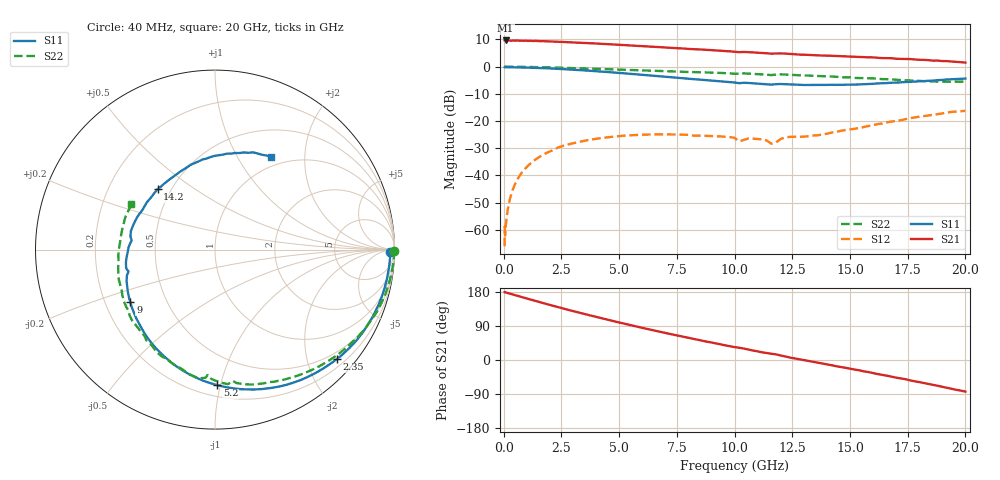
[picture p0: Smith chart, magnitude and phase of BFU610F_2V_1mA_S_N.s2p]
! Filename:  P:\Prog\Test\Noise\ATS_data\Testdata_Net\SplitFiles\BFU610_2W_A5_HighFreq_2V_1mA_D.s2p
! Date/Time: Wed 10/Aug/2011 16:55:42
! BFU610_2W_A5_HighFreq_2V_1mA_10mA_Bias1_R.s2p
! MDIF S-parameter v. bias file
! BFU610_2W_A5_HighFreq_2V_1mA_10mA
! Date/time Mon Aug 08 14:20:39 2011
! bias mode 1
! bias variable = I_out
! VAR bias_var= 1
! VAR V_out= 2.0002
! VAR I_out= 1.0000
! VAR V_in= 0.8491
! VAR I_in= 0.0074
! Device data file deembeded for feedlines and parallel
! Original file: \SplitFiles\BFU610_2W_A5_HighFreq_2V_1mA_R.s2p
! Feed-files: PR003V01_101208_Feed1.s2p, PR003V01_101208_Feed2.s2p
! Parallel-file: PR003V01_101208_Par.s2p
# MHz S MA R 50
!  Freq-MHz  S11-mag  S11-arg  S21-mag  S21-arg  S12-mag  S12-arg  S22-mag  S22-arg
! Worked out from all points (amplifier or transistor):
!   167 points, 40 MHz to 20 GHz, reference 50 ohm
!   highest |S21| = 9.6 dB at 80 MHz (marker M1)
!   |S21| within 3 dB of that: start of sweep to 7.847 GHz
!   unconditionally stable (mu >= 1): 7.79 GHz to end of sweep
!   at 550 MHz: K = -0.01, MSG = 25.9 dB, |S12| = -42.2 dB
!   at 4.2 GHz: K = 0.41, MSG = 17.4 dB, |S12| = -26.3 dB
!   at 20 GHz: K = 1.15, MAG = 6.5 dB, |S12| = -16.2 dB
!   lowest NFmin = 0.80 dB at 400 MHz
!   S11 on the Smith chart (normalised r, x): 40 MHz: 66, -35; 2.35 GHz: 0.35, -2.56; 5.2 GHz: 0.28, -0.98; 9 GHz: 0.31, -0.26; 14.2 GHz: 0.42, +0.36; 20 GHz: 0.86, +1.40
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40  0.9765 -0.7  3.029 179.2  0.0005006 90.2  0.9976 -0.3
50  0.971 -0.7  3.016 179.3  0.001165 82.7  0.9981 -0.5
60  0.9791 -0.9  3.024 178.5  0.0007824 78.1  0.9983 -0.6
80  0.9763 -1.4  3.033 178.4  0.00103 90.7  0.9981 -0.8
140  0.9761 -2.5  3.02 177.4  0.001852 91.5  0.9979 -1.4
280  0.9748 -5.1  3.017 174.9  0.003854 90.3  0.9973 -2.8
700  0.9689 -12.7  2.998 167.6  0.009996 83.8  0.9933 -7.0
1350  0.9521 -24.4  2.98 156.3  0.01924 74.1  0.983 -13.3
2350  0.9123 -42.0  2.876 139.6  0.03263 61.5  0.9593 -22.8
3400  0.8597 -59.7  2.738 122.9  0.04252 47.7  0.9304 -32.0
4300  0.8087 -74.5  2.627 109.3  0.04915 37.8  0.9039 -39.4
5200  0.755 -89.1  2.494 96.3  0.05376 29.0  0.8772 -46.5
6800  0.6629 -114.3  2.279 74.1  0.05693 15.3  0.8324 -58.7
9000  0.5553 -148.0  2.012 46.2  0.05305 4.3  0.7786 -74.8
10200  0.4972 -165.8  1.847 32.4  0.04217 -2.5  0.7389 -82.3
11600  0.4669 173.7  1.734 16.4  0.03821 5.7  0.7002 -93.4
12000  0.4799 167.5  1.753 11.9  0.04689 20.3  0.7216 -96.7
13400  0.4623 145.1  1.626 -4.7  0.05416 18.8  0.6775 -110.5
14200  0.4641 133.5  1.583 -13.7  0.06151 22.4  0.6598 -118.5
16800  0.5067 98.0  1.43 -44.0  0.09795 16.5  0.5834 -150.6
18400  0.5499 78.3  1.316 -63.5  0.1269 4.9  0.5395 -176.6
20000  0.6044 58.6  1.189 -83.4  0.1543 -11.2  0.5299 151.7
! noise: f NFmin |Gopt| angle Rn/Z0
400  0.8033  0.7893  3.377  0.7168
700  0.8406  0.7691  7.269  0.7306
1150  0.8961  0.7445  12.99  0.743
1650  0.9568  0.7232  19.09  0.7462
2100  1.011  0.7078  24.3  0.7405
2600  1.07  0.6929  29.76  0.7259
3500  1.174  0.6668  38.85  0.6812
4400  1.276  0.6356  47.37  0.6194
5600  1.407  0.5797  59.06  0.5232
8000  1.654  0.4482  94.3  0.3485
